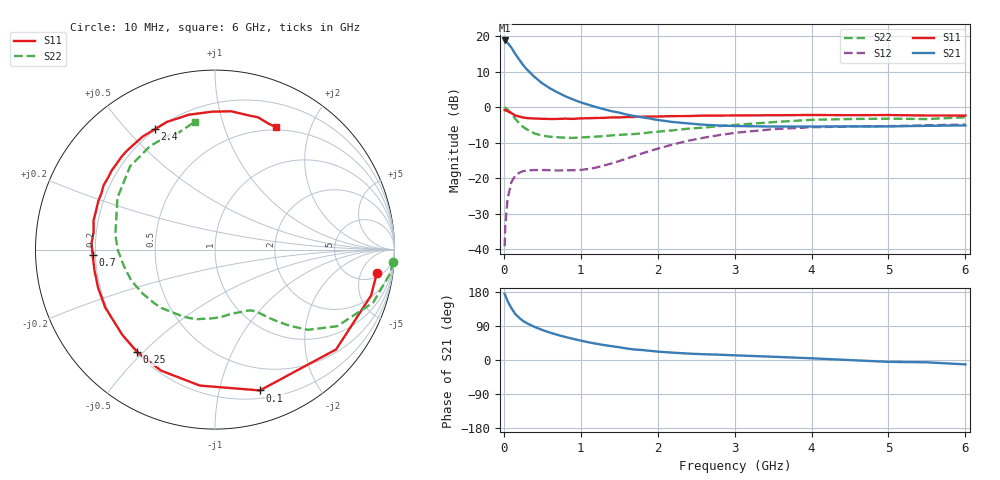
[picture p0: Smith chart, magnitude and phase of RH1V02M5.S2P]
! SIEMENS Small Signal Semiconductors
! BFR106
! Si NPN RF Bipolar Junction Transistor in SOT23
! VCE = 1 V  IC = 2.5 mA
! Common Emitter S-Parameters:  August  1996
# GHz  S  MA  R  50
!  f  S11  S21  S12  S22
! GHz  MAG  ANG  MAG  ANG  MAG  ANG  MAG  ANG
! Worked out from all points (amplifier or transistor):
!   36 points, 10 MHz to 6 GHz, reference 50 ohm
!   highest |S21| = 18.8 dB at 10 MHz (marker M1)
!   |S21| within 3 dB of that: start of sweep to 126 MHz
!   unconditionally stable (mu >= 1): 718.5 MHz to end of sweep
!   at 250 MHz: K = 0.37, MSG = 15.0 dB, |S12| = -18.1 dB
!   at 1.4 GHz: K = 1.29, MAG = 4.1 dB, |S12| = -15.9 dB
!   at 6 GHz: K = 1.03, MAG = -1.1 dB, |S12| = -4.9 dB
!   S11 on the Smith chart (normalised r, x): 10 MHz: 6, -10; 100 MHz: 0.27, -1.33; 250 MHz: 0.20, -0.48; 700 MHz: 0.19, -0.02; 2.4 GHz: 0.20, +0.60; 6 GHz: 0.47, +1.52
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0.01  0.9114 -8.2  8.704 174.3  0.011 85.8  0.9941 -3.9
0.02  0.9064 -16.4  8.61 169.9  0.0223 82.7  0.9849 -7.8
0.05  0.8744 -39.5  8.052 154.9  0.0522 68.2  0.9295 -18.5
0.1  0.8236 -72.3  6.841 136.2  0.0887 52.5  0.8035 -32.1
0.15  0.7623 -96.4  5.593 121.2  0.1085 40.9  0.6825 -40.9
0.2  0.7382 -114.1  4.683 111.4  0.1191 34.2  0.5938 -45.6
0.25  0.7157 -127.3  3.931 103.0  0.1251 29.3  0.5267 -49.2
0.3  0.702 -137.2  3.388 97.1  0.1281 26.3  0.4857 -51.6
0.4  0.6915 -152.1  2.66 87.3  0.13 23.0  0.4259 -55.4
0.5  0.6853 -162.1  2.165 79.2  0.1301 21.7  0.3961 -58.8
0.6  0.6815 -170.6  1.842 72.3  0.1293 22.1  0.3829 -62.8
0.7  0.6825 -177.5  1.61 66.1  0.1282 23.7  0.3764 -67.5
0.9  0.6829 171.8  1.284 55.8  0.129 29.6  0.3694 -77.0
1.1  0.6975 161.7  1.081 46.8  0.1344 37.3  0.3792 -87.9
1.6  0.725 142.5  0.784 30.2  0.189 51.8  0.4138 -115.7
2.2  0.7477 122.6  0.617 19.3  0.2987 50.7  0.472 -148.8
2.4  0.7495 116.6  0.59 16.9  0.3368 47.7  0.4975 -159.9
3  0.7656 100.9  0.542 12.3  0.4339 35.8  0.5611 171.8
3.5  0.7685 91.2  0.533 8.6  0.4898 25.6  0.6155 152.0
4.5  0.7707 77.2  0.536 -0.2  0.5339 7.8  0.681 122.1
5.5  0.7627 67.1  0.546 -6.1  0.5547 -2.1  0.6796 108.0
6  0.7618 63.4  0.553 -11.6  0.5693 -9.0  0.7212 99.0
